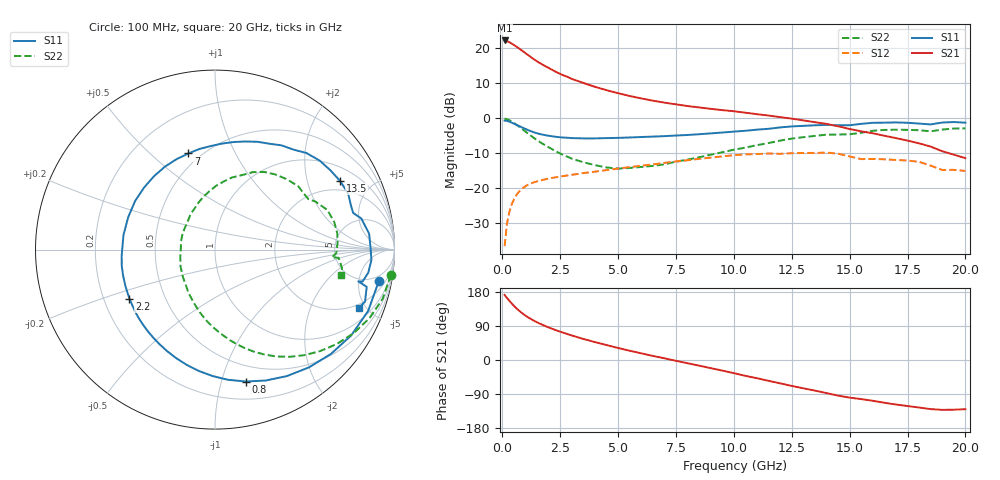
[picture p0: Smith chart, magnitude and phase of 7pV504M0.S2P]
! Infineon Technologies  Discrete & RF Semiconductors
! bfp620
! VCE = 0.50 V,  IC =  4.0 mA
! Common Emitter S-Parameters:  Sep 2002
# GHz  S  MA  R  50
!  f  S11  S21  S12  S22
! GHz  MAG  ANG  MAG  ANG  MAG  ANG  MAG  ANG
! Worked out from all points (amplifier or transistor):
!   59 points, 100 MHz to 20 GHz, reference 50 ohm
!   highest |S21| = 22.3 dB at 100 MHz (marker M1)
!   |S21| within 3 dB of that: start of sweep to 872 MHz
!   unconditionally stable (mu >= 1): 5.007 GHz to 10.91 GHz; 17.01 GHz to end of sweep
!   at 1 GHz: K = 0.29, MSG = 19.0 dB, |S12| = -19.4 dB
!   at 5.5 GHz: K = 1.04, MAG = 9.0 dB, |S12| = -14.0 dB
!   at 20 GHz: K = 1.83, MAG = -3.4 dB, |S12| = -15.1 dB
!   S11 on the Smith chart (normalised r, x): 100 MHz: 3.50, -9.05; 800 MHz: 0.35, -1.20; 2.2 GHz: 0.31, -0.24; 7 GHz: 0.43, +0.67; 13.5 GHz: 1.54, +3.21; 20 GHz: 1.74, -4.52
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0.1  0.929 -11.0  13.01 171.7  0.0148 81.7  0.9906 -8.2
0.2  0.9193 -21.8  12.71 163.9  0.0308 77.6  0.9732 -16.4
0.3  0.897 -32.2  12.27 156.6  0.0451 72.0  0.9415 -24.0
0.4  0.869 -42.0  11.76 149.7  0.0578 66.5  0.9019 -31.1
0.5  0.8396 -51.4  11.22 143.2  0.069 61.6  0.8586 -37.8
0.6  0.8105 -60.4  10.67 137.1  0.0788 57.1  0.8142 -44.0
0.8  0.7552 -76.7  9.591 126.3  0.0948 49.4  0.7274 -55.2
1  0.7047 -91.1  8.57 117.2  0.1067 43.3  0.6468 -64.7
1.1  0.6818 -97.7  8.098 113.2  0.1114 40.7  0.6097 -69.0
1.4  0.6256 -115.2  6.879 102.7  0.1224 34.4  0.514 -80.3
1.6  0.5989 -125.2  6.241 96.6  0.128 31.3  0.4634 -86.9
1.8  0.5789 -134.2  5.714 91.1  0.1329 28.7  0.4216 -93.1
2.2  0.5498 -150.1  4.849 81.3  0.1412 24.5  0.3543 -104.6
2.8  0.5275 -170.0  3.942 68.8  0.1519 19.7  0.2837 -121.2
3.5  0.5164 171.0  3.209 55.6  0.1644 15.0  0.2355 -139.3
5  0.5252 138.7  2.289 31.7  0.1909 6.2  0.1906 179.3
7  0.5558 105.5  1.677 4.5  0.2302 -6.4  0.2197 133.4
8.5  0.5919 86.3  1.432 -14.9  0.263 -17.8  0.2768 109.6
10.5  0.6633 62.8  1.204 -41.8  0.3042 -37.5  0.381 83.0
13.5  0.795 28.8  0.881 -80.7  0.3201 -68.1  0.5602 44.4
17  0.8734 -3.8  0.521 -117.4  0.2536 -99.0  0.6871 7.6
20  0.8666 -21.9  0.269 -129.8  0.1767 -114.3  0.7184 -11.3
